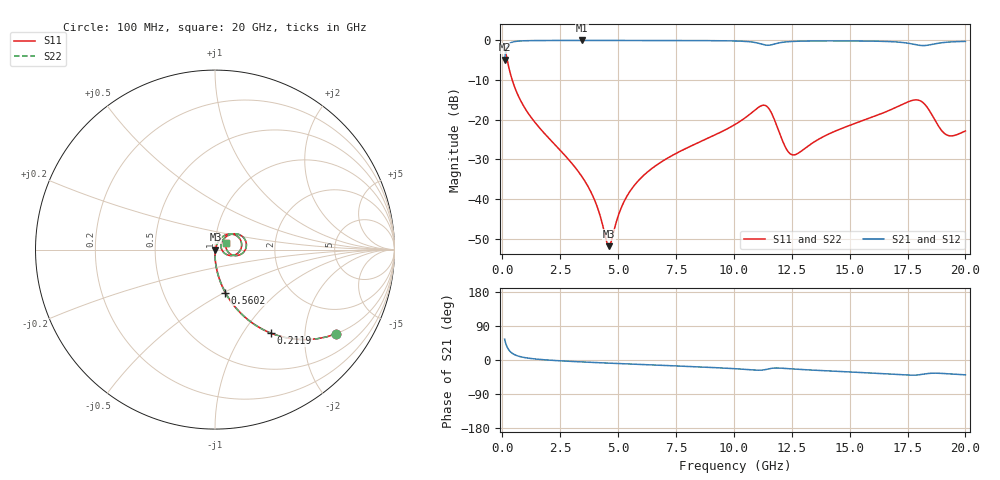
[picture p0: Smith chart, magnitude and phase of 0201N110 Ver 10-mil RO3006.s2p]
# GHz S MA R 50
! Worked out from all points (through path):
!   1601 points, 100 MHz to 20 GHz, reference 50 ohm
!   highest |S21| = -0.02 dB at 3.446 GHz (marker M1); lowest = -4.9 dB at 100 MHz (marker M2)
!   group delay of S21, straight-line fit = 6.8 ps
!   lowest |S11| = -51.9 dB at 4.602 GHz (marker M3), VSWR 1.01, Z = 50.3 - j0.0441 ohm
!   |S11| at or under -10 dB: 428.7 MHz to end of sweep
!   |S22| runs from -51.9 to -1.7 dB; largest |S21 - S12| = 0
!   S11 on the Smith chart (normalised r, x): 100 MHz: 0.99, -2.87; 211.9 MHz: 0.99, -1.35; 560.2 MHz: 0.99, -0.51; 20 GHz: 1.13, +0.08
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0.1  0.8214 -34.9  0.5698 55.0  0.5698 55.0  0.8214 -34.9
0.2119375  0.5614 -56.1  0.8267 33.8  0.8267 33.8  0.5614 -56.1
0.34875  0.3801 -68.2  0.9241 21.7  0.9241 21.7  0.3801 -68.2
0.5601875  0.2458 -76.6  0.9684 13.2  0.9684 13.2  0.2458 -76.6
1.306437  0.1013 -85.8  0.9935 3.5  0.9935 3.5  0.1013 -85.8
3.420812  0.01952 -88.7  0.9976 -5.1  0.9976 -5.1  0.01952 -88.7
3.445688  0.01905 -88.6  0.9976 -5.1  0.9976 -5.1  0.01905 -88.6
4.017812  0.009224 -81.9  0.9975 -6.7  0.9975 -6.7  0.009224 -81.9
4.602375  0.002547 -9.9  0.9973 -8.3  0.9973 -8.3  0.002547 -9.9
5.087438  0.007145 58.2  0.9971 -9.5  0.9971 -9.5  0.007145 58.2
5.435688  0.01153 65.4  0.997 -10.4  0.997 -10.4  0.01153 65.4
6.741625  0.02779 69.3  0.9961 -13.7  0.9961 -13.7  0.02779 69.3
10.05  0.08701 58.4  0.9829 -23.0  0.9829 -23.0  0.08701 58.4
11.33106  0.1519 13.0  0.8766 -25.7  0.8766 -25.7  0.1519 13.0
11.60469  0.1248 -10.7  0.8771 -22.2  0.8771 -22.2  0.1248 -10.7
12.42556  0.03736 1.8  0.9657 -23.1  0.9657 -23.1  0.03736 1.8
13.37081  0.05024 45.1  0.9827 -26.6  0.9827 -26.6  0.05024 45.1
16.69162  0.1304 42.0  0.9664 -37.0  0.9664 -37.0  0.1304 42.0
17.97269  0.1764 7.5  0.8703 -39.2  0.8703 -39.2  0.1764 7.5
18.3085  0.1488 -9.6  0.8642 -36.2  0.8642 -36.2  0.1488 -9.6
19.14181  0.06562 -1.4  0.9448 -35.9  0.9448 -35.9  0.06562 -1.4
20  0.07219 29.8  0.9713 -39.1  0.9713 -39.1  0.07219 29.8
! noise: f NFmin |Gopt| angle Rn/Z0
0.1  0.0006424  0.9333  0.3781  0.002143
2.301  0.003995  0.7731  4.245  0.003589
4.515  0.006702  0.74  8.143  0.005139
6.729  0.009464  0.7282  12.03  0.006854
8.943  0.01442  0.7595  15.92  0.01192
11.14  0.06347  0.9258  19.93  0.1839
13.36  0.02879  0.816  23.78  0.03133
15.57  0.02866  0.7889  27.53  0.02641
17.79  0.08546  0.914  31.46  0.203
20  0.04477  0.8252  35.19  0.04896
